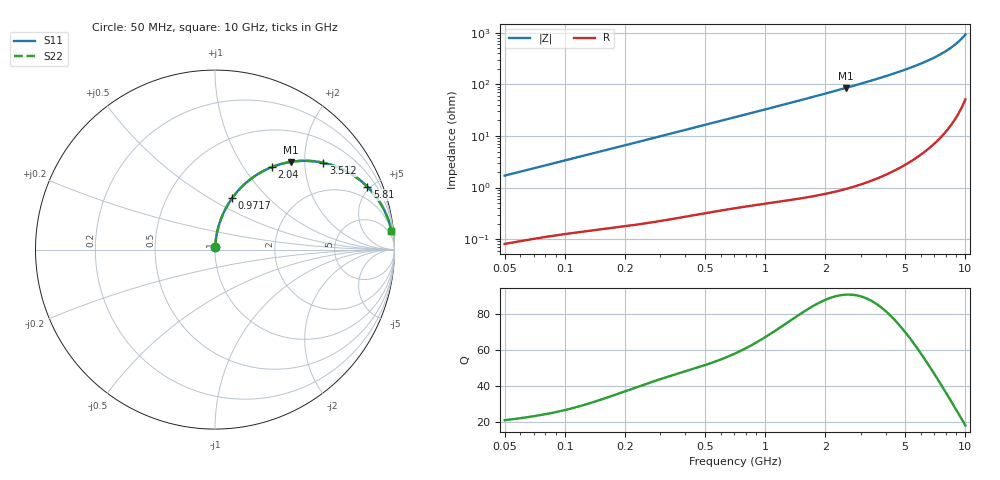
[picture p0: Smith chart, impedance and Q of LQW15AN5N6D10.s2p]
!Murata Part Number: LQW15AN5N6D10
!These Parameters are Measured in Series Mode Connection
!  o--[Z]--o
!Port1  Port2
!  o-------o
!Freq. Start=50[MHz] Stop=10[GHz], 401[Steps]
# Hz S RI R 50
!Freq.(Hz)	S 11(Real)	S 11(Imag)	S 21(Real)	S 21(Imag)	S 12(Real)	S 12(Imag)	S 22(Real)	S 22(Imag)
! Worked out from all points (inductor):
!   401 points, 50 MHz to 10 GHz, reference 50 ohm
!   read as one part in series: L = 5.39 nH near 51.34 MHz
!   highest Q = 91 at 2.522 GHz (marker M1), where L = 5.38 nH
!   S11 on the Smith chart (normalised r, x): 50 MHz: 1.00, +0.03; 971.7 MHz: 1.01, +0.64; 2.04 GHz: 1.02, +1.36; 3.512 GHz: 1.03, +2.47; 5.81 GHz: 1.08, +4.83; 10 GHz: 2, +19
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5e7  0.0011 0.017  0.9989 -0.017  0.9989 -0.017  0.0011 0.017
1.214486e8  0.00302 0.0403  0.997 -0.0403  0.997 -0.0403  0.00302 0.0403
1.956524e8  0.00591 0.0643  0.9941 -0.0643  0.9941 -0.0643  0.00591 0.0643
2.949953e8  0.0115 0.0959  0.9885 -0.0959  0.9885 -0.0959  0.0115 0.0959
4.628099e8  0.0254 0.1477  0.9746 -0.1477  0.9746 -0.1477  0.0254 0.1477
7.071068e8  0.0543 0.2182  0.9457 -0.2182  0.9457 -0.2182  0.0543 0.2182
9.717327e8  0.0955 0.2865  0.9045 -0.2865  0.9045 -0.2865  0.0955 0.2865
1.300479e9  0.1576 0.3578  0.8424 -0.3578  0.8424 -0.3578  0.1576 0.3578
1.717543e9  0.2466 0.4252  0.7534 -0.4252  0.7534 -0.4252  0.2466 0.4252
2.040286e9  0.3181 0.4601  0.6819 -0.4601  0.6819 -0.4601  0.3181 0.4601
2.521925e9  0.4219 0.4884  0.5781 -0.4884  0.5781 -0.4884  0.4219 0.4884
2.99582e9  0.5151 0.4943  0.4849 -0.4943  0.4849 -0.4943  0.5151 0.4943
3.511936e9  0.6037 0.4834  0.3963 -0.4834  0.3963 -0.4834  0.6037 0.4834
4.171863e9  0.6969 0.4534  0.3031 -0.4534  0.3031 -0.4534  0.6969 0.4534
4.955797e9  0.7818 0.406  0.2182 -0.406  0.2182 -0.406  0.7818 0.406
5.809576e9  0.8493 0.3496  0.1507 -0.3496  0.1507 -0.3496  0.8493 0.3496
6.901252e9  0.9084 0.2783  0.0916 -0.2783  0.0916 -0.2783  0.9084 0.2783
7.983737e9  0.9462 0.2123  0.0538 -0.2123  0.0538 -0.2123  0.9462 0.2123
8.876195e9  0.9668 0.1623  0.0332 -0.1623  0.0332 -0.1623  0.9668 0.1623
9.359165e9  0.9749 0.1368  0.0251 -0.1368  0.0251 -0.1368  0.9749 0.1368
9.738562e9  0.98 0.1176  0.02 -0.1176  0.02 -0.1176  0.98 0.1176
1e10  0.983 0.1047  0.017 -0.1047  0.017 -0.1047  0.983 0.1047
